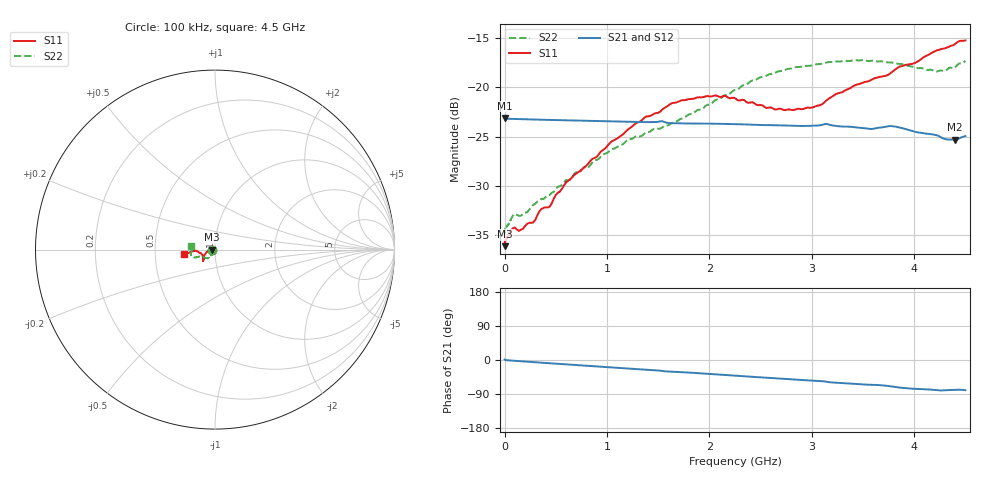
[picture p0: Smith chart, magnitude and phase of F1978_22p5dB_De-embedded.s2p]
! Integrated Device Technology
! Corporate Headquarters
! 6024 Silver Creek Valley Road
! San Jose, CA 95138  USA
! Phone:  1-408-284-8200
! Toll Free:  1-800-223-1366
! Webpage:  http://www.idt.com/
! Timing and RF Division
! 515 Groton Road, Suite 102
! Westford, MA 01886-6024
! Device:  F1978
! Description: 6-bit, 75 ohm, 0.5 dB Digital Step Attenuator
! Frequency:  5.0 MHz -  3.00 GHz
! Package:  4x4 mm QFN Plastic Package: 20 pin
! Ports:  2 RF, 11 DC
!  Pin  1  = D5 (16 dB)
!  Pin  2  = RF1  =  Port 1
!  Pin  3  = Serial Data In (DATA)
!  Pin  4  = Serial Clock (CLK)
!  Pin  5  = Serial Latch Enable (LE)
!  Pin  6  = VDD
!  Pin  7  = NC
!  Pin  8  = NC
!  Pin  9  = NC
!  Pin 10  = GND
!  Pin 11  = GND
!  Pin 12  = NC
!  Pin 13  = VMODE
!  Pin 14  = RF2  =  Port 2
!  Pin 15  = D4 (8 dB)
!  Pin 16  = D3 (4 dB)
!  Pin 17  = D2 (2 dB)
!  Pin 18  = NC
!  Pin 19  = D1 (1 dB)
!  Pin 20  = D0 (0.5 dB)
! State:  45
! Atten State:  22.5 dB
! Voltage:  +3.30 Volts
! Current:  0.562 mA
! Data:  The device was measured on a F1975 evaluation board which has
!  individual transmission lines to the RF pins.  Data was collected
!  using a calibrated network analyzer.  The evaluation board was
!  de-embedded using Automatic Fixture Removal (AFR).
!  The reference plane is the edge of the package pin.
! Misc:
!  Action Tracker AT0416
! Date Measured:  2018-02-08
! Date:  2018-03-26  MJV
! Note:
!  Integrated Device Technology supplies this data as a sample of measured
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# GHz S dB R 75
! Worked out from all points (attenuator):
!   291 points, 100 kHz to 4.5 GHz, reference 75 ohm
!   highest |S21| = -23.11 dB at 100 kHz (marker M1); lowest = -25.3 dB at 4.4 GHz (marker M2)
!   lowest |S11| = -36.1 dB at 100 kHz (marker M3), VSWR 1.03, Z = 72.7 - j0.0119 ohm
!   |S11| at or under -10 dB: start of sweep to end of sweep
!   |S22| runs from -35.0 to -17.2 dB; largest |S21 - S12| = 0.00016
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0.0001  -36.15 -179.7  -23.11 1.2  -23.12 1.2  -34.99 -179.1
0.002  -35.70 -178.4  -23.15 0.8  -23.16 0.9  -34.62 -176.9
0.011  -35.48 -178.2  -23.19 -0.4  -23.18 -0.4  -34.20 -175.6
0.1  -34.26 -175.4  -23.21 -2.1  -23.21 -2.2  -32.87 -161.7
0.16  -34.46 -177.7  -23.24 -3.3  -23.23 -3.3  -33.04 -154.4
0.28  -33.73 179.8  -23.27 -5.6  -23.27 -5.6  -31.95 -144.7
0.36  -32.37 179.9  -23.29 -7.1  -23.29 -7.1  -31.33 -137.0
0.44  -32.14 -179.5  -23.31 -8.6  -23.31 -8.6  -30.94 -131.3
0.6  -29.66 -175.8  -23.35 -11.6  -23.35 -11.6  -29.42 -126.5
0.76  -28.30 -169.0  -23.39 -14.5  -23.38 -14.5  -28.28 -123.8
1.28  -23.67 -152.8  -23.51 -23.8  -23.51 -23.8  -24.99 -123.1
1.52  -22.47 -144.7  -23.45 -28.1  -23.45 -28.1  -24.19 -129.7
1.64  -21.59 -142.6  -23.64 -30.6  -23.64 -30.6  -23.61 -133.5
1.88  -21.03 -139.0  -23.68 -34.5  -23.68 -34.5  -22.32 -144.6
2.26  -21.17 -138.1  -23.73 -41.4  -23.73 -41.4  -20.25 -155.4
2.64  -22.25 -147.5  -23.85 -48.2  -23.85 -48.2  -18.54 -158.6
3.02  -22.00 -163.9  -23.89 -54.5  -23.88 -54.5  -17.72 -160.9
3.42  -19.80 -175.3  -24.06 -63.3  -24.05 -63.3  -17.21 -166.5
3.76  -18.63 -175.8  -23.94 -69.1  -23.94 -69.1  -17.46 -173.0
4.2  -16.34 -172.7  -24.83 -79.0  -24.82 -79.0  -18.39 175.3
4.4  -15.59 -170.6  -25.32 -78.9  -25.32 -78.9  -17.98 171.9
4.5  -15.23 -172.5  -24.95 -79.7  -24.95 -79.7  -17.29 170.4
